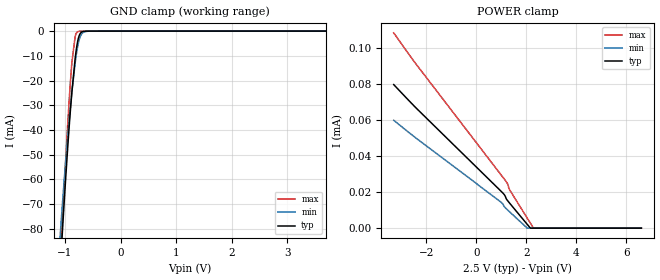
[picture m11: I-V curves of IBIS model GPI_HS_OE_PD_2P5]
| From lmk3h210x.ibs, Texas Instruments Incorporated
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[Model]   GPI_HS_OE_PD_2P5
Model_type   Input
Vinl = 0.65
Vinh = 1.15
|   typ   min   max
C_comp   0.55pF   0.44pF   0.66pF
[Voltage Range]   2.5   2.375   2.625
[Temperature Range]   45   125   -40
[Power Clamp Reference]   2.5   2.375   2.625
[GND Clamp Reference]   0   0   0
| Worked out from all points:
|   GND clamp passes 1 mA (typ) near -0.73 V on its own axis
[GND Clamp]
|   Voltage   I(typ)   I(min)   I(max)
-3.3V     -1.046A    -940.8mA   -1.157A
-1.142V   -118.3mA   -101.5mA   -119.6mA
-1.073V   -91.27mA   -78.48mA   -88.66mA
-1.043V   -80.01mA   -69.14mA   -75.72mA
-943.8mV  -45.02mA   -41.08mA   -35.24mA
-904.2mV  -32.76mA   -31.3mA    -21.3mA
-874.5mV  -24.5mA    -24.51mA   -12.52mA
-815.1mV  -10.86mA   -12.73mA   -2.013mA
-765.6mV  -3.574mA   -5.611mA   -223.9uA
-696.3mV  -364.2uA   -1.075mA   -30.26uA
-557.7mV  -16.92uA   -43.6uA    -19.9uA
6.6V      0A         0A         0A
[POWER Clamp]
|   Voltage   I(typ)   I(min)   I(max)
-3.3V     79.74uA    59.93uA    108.4uA
-2.399V   66.65uA    49.93uA    90.99uA
986.7mV   20.57uA    14.44uA    29.67uA
1.125V    18.5uA     11.88uA    27.15uA
1.195V    16.48uA    10.86uA    25.87uA
1.254V    15.25uA    10.08uA    24.48uA
1.304V    14.4uA     9.442uA    22.18uA
1.343V    13.73uA    8.932uA    21.1uA
2.036V    2.137uA    41.85nA    5.635uA
2.155V    151.4nA    0A         2.99uA
2.284V    0A         0A         125.3nA
6.6V      0A         0A         0A
